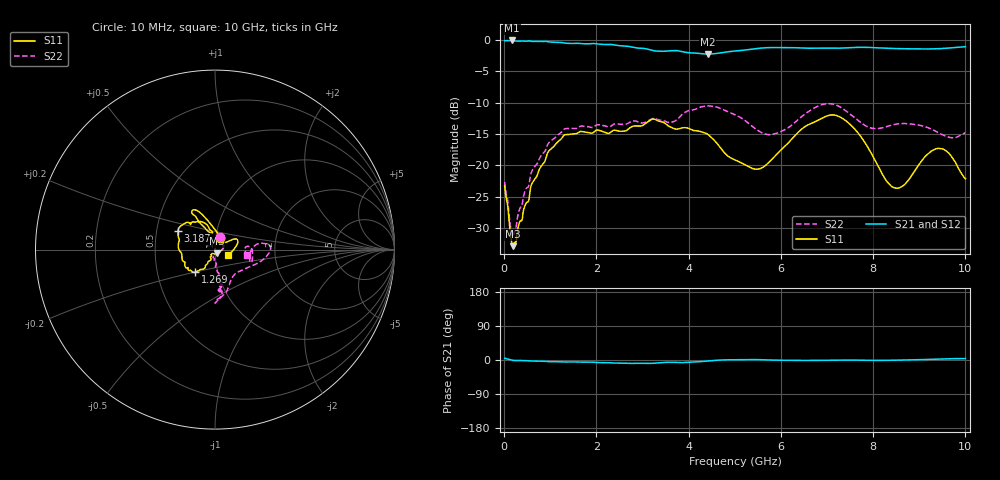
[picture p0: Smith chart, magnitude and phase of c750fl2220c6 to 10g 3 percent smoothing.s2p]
!Agilent Technologies,N5234A,MY52241123,A.10.00.00
!Agilent N5234A: A.10.00.00
!Date: Tuesday, April 23, 2019 10:49:05
!Correction: S11(Full 2 Port(1,2))
!S21(Full 2 Port(1,2))
!S12(Full 2 Port(1,2))
!S22(Full 2 Port(1,2))
!S2P File: Measurements: S11, S21, S12, S22:
# Hz S  dB  R 50
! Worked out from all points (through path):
!   1001 points, 10 MHz to 10 GHz, reference 50 ohm
!   highest |S21| = -0.10 dB at 169.8 MHz (marker M1); lowest = -2.3 dB at 4.416 GHz (marker M2)
!   lowest |S11| = -32.9 dB at 189.8 MHz (marker M3), VSWR 1.05, Z = 51 - j2.07 ohm
!   |S11| at or under -10 dB: start of sweep to end of sweep
!   |S22| runs from -31.3 to -10.2 dB; largest |S21 - S12| = 0.00096
!   S11 on the Smith chart (normalised r, x): 10 MHz: 1.04, +0.13; 1.269 GHz: 0.78, -0.20; 3.187 GHz: 0.65, +0.14; 10 GHz: 1.15, -0.08
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1e7  -23.24 68.0  -0.14 4.7  -0.14 4.7  -22.65 67.2
1.6984e8  -32.62 -49.3  -0.10 -0.5  -0.09 -0.5  -31.14 -37.5
1.8982e8  -32.86 -62.8  -0.11 -0.9  -0.10 -0.9  -31.30 -49.5
6.2938e8  -22.56 -119.0  -0.25 -2.6  -0.25 -2.6  -20.53 -88.5
1.26874e9  -15.45 -131.4  -0.45 -5.2  -0.44 -5.2  -14.47 -79.1
1.67833e9  -14.59 -143.2  -0.61 -5.6  -0.61 -5.6  -13.72 -79.3
2.59741e9  -14.54 -173.1  -0.97 -8.3  -0.96 -8.3  -13.45 -83.2
3.18682e9  -12.72 152.9  -1.62 -9.0  -1.62 -9.0  -12.63 -81.1
3.34666e9  -12.93 141.7  -1.80 -7.4  -1.80 -7.4  -12.74 -84.7
4.41559e9  -15.05 117.6  -2.27 -2.7  -2.27 -2.7  -10.51 -89.9
5.005e9  -19.13 103.1  -1.79 0.8  -1.79 0.8  -11.93 -77.8
5.46454e9  -20.60 100.7  -1.39 1.1  -1.39 1.1  -14.25 -63.1
5.77423e9  -19.25 110.7  -1.23 -0.0  -1.23 -0.0  -15.10 -48.8
6.67333e9  -13.26 120.6  -1.34 -0.9  -1.33 -1.0  -11.06 -9.9
7.1029e9  -11.96 119.6  -1.32 -0.7  -1.32 -0.8  -10.20 2.9
7.41259e9  -12.91 112.5  -1.28 -0.2  -1.27 -0.2  -11.32 7.4
7.92208e9  -17.57 96.6  -1.21 -0.9  -1.21 -1.0  -13.97 -2.3
8.34166e9  -22.92 61.1  -1.35 -0.8  -1.35 -0.8  -13.70 -18.9
8.64136e9  -23.27 36.1  -1.41 -0.2  -1.40 -0.2  -13.33 -17.4
9.41059e9  -17.28 23.1  -1.41 2.4  -1.41 2.4  -14.77 5.9
9.65035e9  -18.12 11.7  -1.30 3.4  -1.29 3.3  -15.53 2.5
1e10  -22.12 -24.6  -1.09 3.8  -1.09 3.8  -14.80 -8.9
